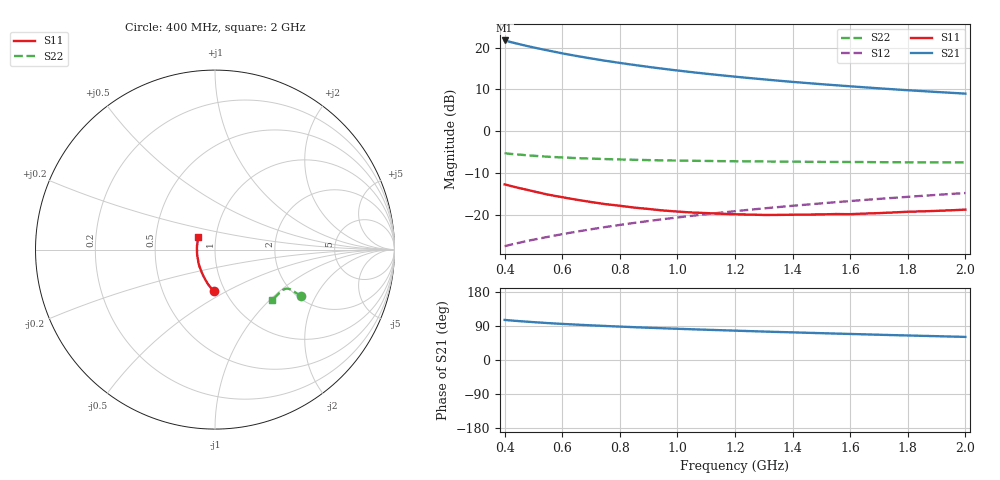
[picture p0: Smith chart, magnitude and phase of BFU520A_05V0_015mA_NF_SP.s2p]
! Filename:  P:\Prog\Test\Noise\ATS_data\Testdata_Net\06 Compressed Noise after Statistics\BFU520A_APG2013_30_A05_05p0V_015mA_NF_CM01_D.sf
! Date/Time: Wed 24/Apr/2013 20:06:18
! BFU520A_APG2013_30_A05_05p0V_1to20mA_NF_CM01_Bias7_R.sf
! Noise Parameter Data File
! BFU520A_APG2013_30_A05_05p0V_1to20mA_NF_CM01
! Date/time: Thu Apr 11 01:07:08 2013
! VAR V_out= 5.000000
! VAR I_out= 15.000000
! VAR V_in= 0.846800
! VAR I_in= 0.168650
! Device data file deembeded for feedlines and parallel
! Original file: \06 Compressed Noise after Statistics\BFU520A_APG2013_30_A05_05p0V_015mA_NF_CM01_R.sf
! Feed-files: PR017V01_150413_Feed1.s2p, PR017V01_150413_Feed2.s2p
! Parallel-file: PR017V01_150413_Par.s2p
# MHz S MA R 50
!  Freq-MHz  S11-mag  S11-arg  S21-mag  S21-arg  S12-mag  S12-arg  S22-mag  S22-arg
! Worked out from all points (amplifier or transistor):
!   37 points, 400 MHz to 2 GHz, reference 50 ohm
!   highest |S21| = 21.7 dB at 400 MHz (marker M1)
!   |S21| within 3 dB of that: start of sweep to 594.5 MHz
!   unconditionally stable (mu >= 1): 1.038 GHz to 1.939 GHz
!   at 500 MHz: K = 0.90, MSG = 22.9 dB, |S12| = -25.9 dB
!   at 1.1 GHz: K = 1.00, MAG = 16.5 dB, |S12| = -19.8 dB
!   at 2 GHz: K = 1.00, MSG = 11.9 dB, |S12| = -14.7 dB
!   lowest NFmin = 1.01 dB at 420 MHz
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400  0.2323 -91.6  12.15 105.7  0.04254 71.8  0.5467 -28.3
420  0.2233 -93.8  11.65 104.4  0.04421 71.9  0.538 -28.3
440  0.2143 -96.2  11.21 103.2  0.04584 72.1  0.5303 -28.2
460  0.2068 -98.2  10.78 102.1  0.04751 72.3  0.5234 -28.2
480  0.1995 -100.5  10.39 101.0  0.04916 72.4  0.5164 -28.1
500  0.1922 -102.6  10.02 99.9  0.05082 72.5  0.5109 -28.1
550  0.1756 -107.9  9.233 97.4  0.05491 73.0  0.497 -27.9
600  0.1634 -112.7  8.523 95.3  0.05918 73.2  0.4873 -27.8
650  0.1525 -117.4  7.93 93.3  0.06339 73.4  0.4788 -27.9
700  0.1432 -122.2  7.41 91.5  0.06766 73.7  0.472 -27.9
750  0.1351 -126.7  6.951 89.8  0.07196 73.8  0.466 -28.0
800  0.1291 -131.6  6.552 88.2  0.07628 73.9  0.4613 -28.2
850  0.1229 -136.4  6.194 86.6  0.08059 74.0  0.4568 -28.4
950  0.1135 -145.5  5.581 83.7  0.08928 74.0  0.4501 -29.0
1050  0.1073 -154.1  5.082 81.1  0.09798 73.9  0.4447 -29.8
1150  0.1038 -163.3  4.67 78.6  0.1068 73.7  0.4405 -30.6
1200  0.1023 -167.2  4.489 77.4  0.1113 73.6  0.439 -31.1
1350  0.1004 -179.2  4.023 74.0  0.1246 73.1  0.4353 -32.7
1500  0.1018 169.8  3.652 70.8  0.1379 72.5  0.4312 -34.5
1600  0.1025 164.0  3.445 68.7  0.1471 72.0  0.4299 -35.8
1750  0.1075 154.7  3.172 65.7  0.1605 71.2  0.4275 -37.8
2000  0.1161 142.8  2.817 61.0  0.1833 69.8  0.4248 -41.6
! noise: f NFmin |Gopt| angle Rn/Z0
400  1.064  0.1491  -168.9  0.095
460  1.02  0.1662  -163.1  0.0897
600  1.137  0.1435  -148.9  0.1132
800  1.079  0.1866  -153.7  0.0892
1000  1.1  0.1897  -150.5  0.0931
1200  1.134  0.2026  -143.7  0.0996
1400  1.192  0.2182  -138.8  0.0996
1600  1.173  0.2407  -133.9  0.1004
1800  1.172  0.2713  -129.5  0.1033
2000  1.204  0.2718  -129.6  0.1076
